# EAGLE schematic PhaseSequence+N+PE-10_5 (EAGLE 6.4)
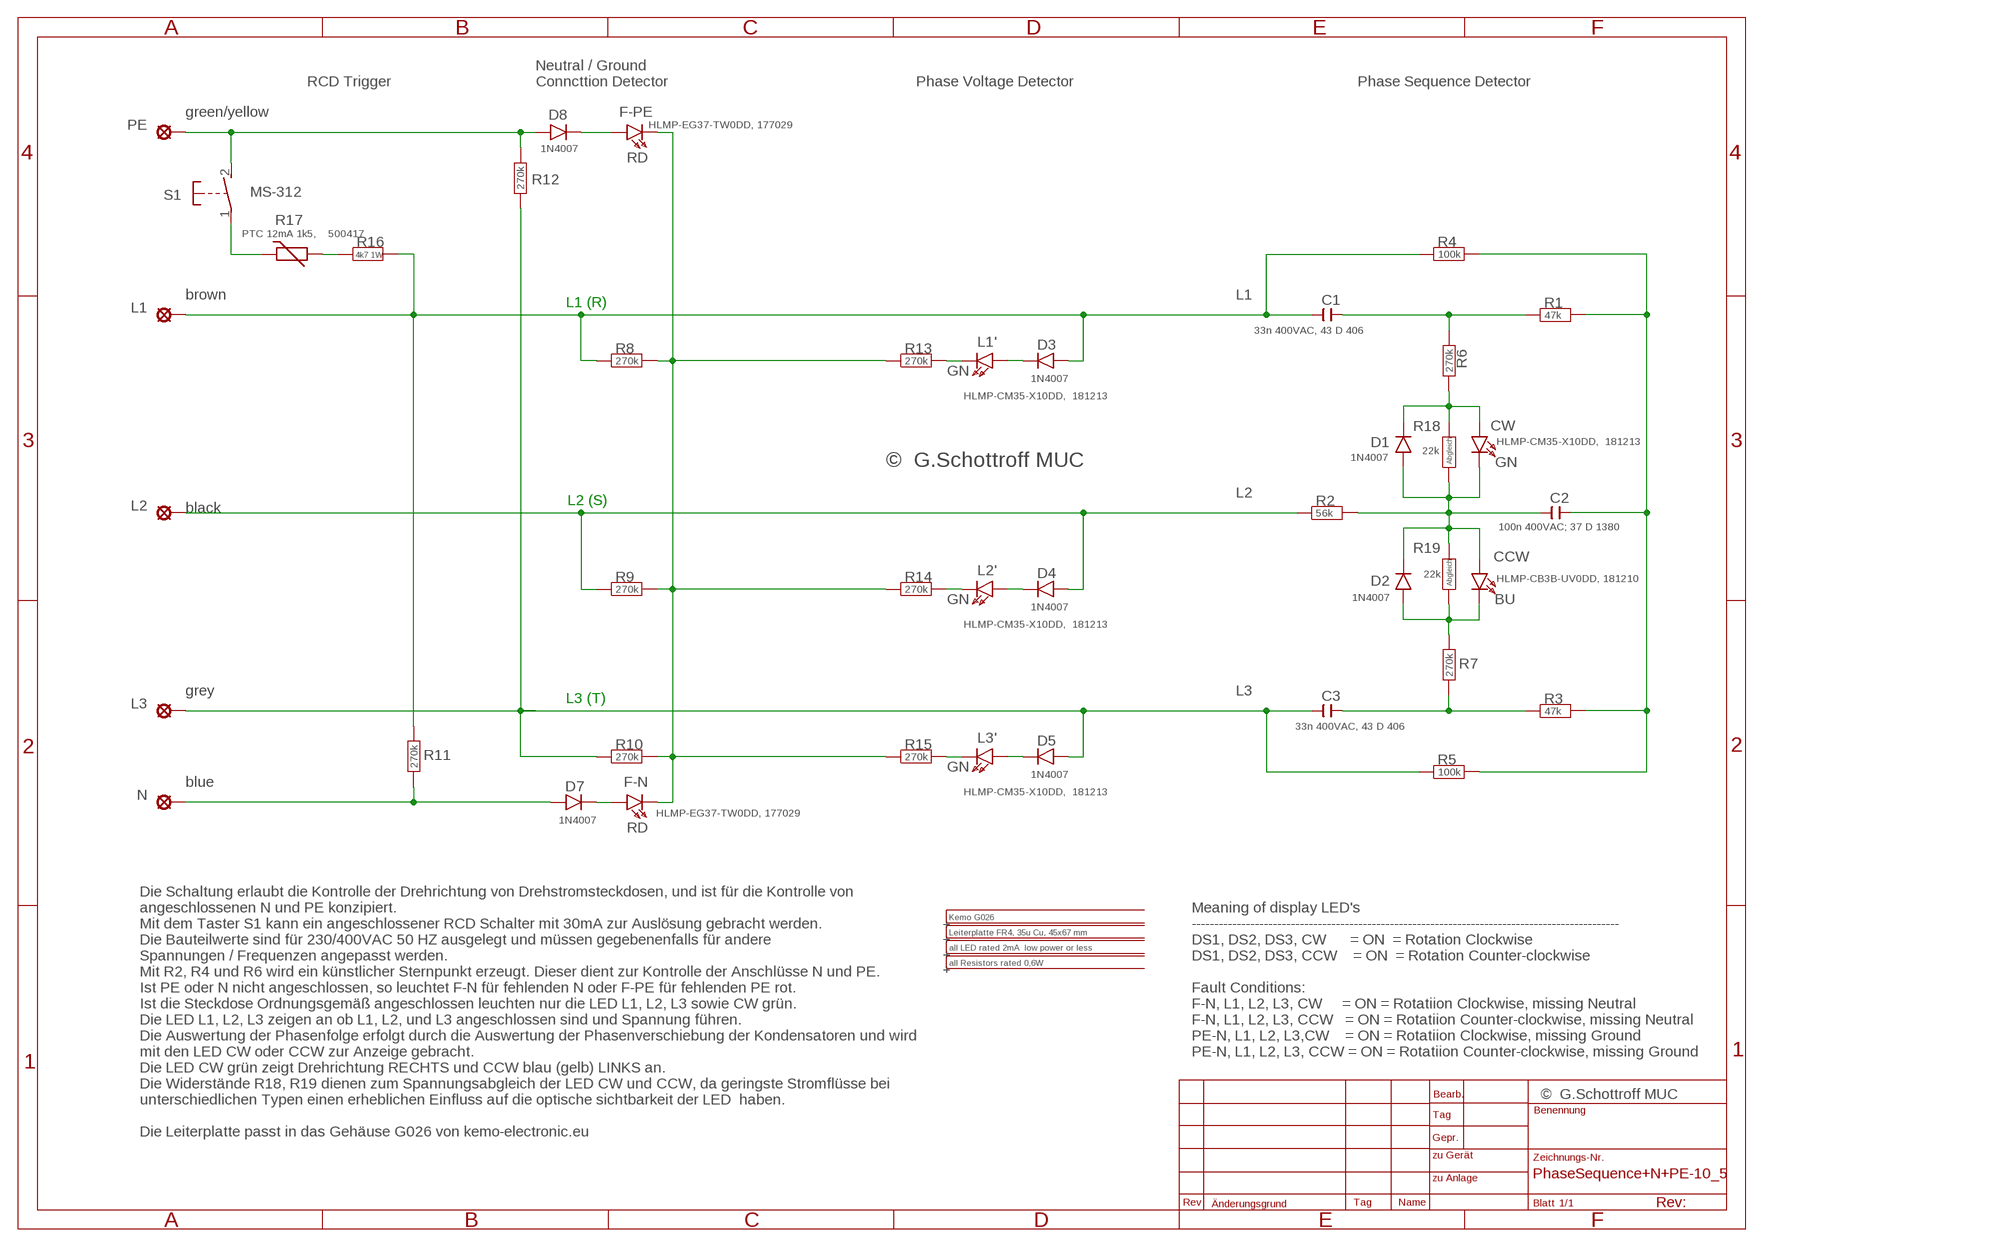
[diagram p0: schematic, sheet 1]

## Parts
C1  33n 400VAC, 43 D 406  C-EU150-064X183  [C150-064X183]
C2  100n 400VAC; 37 D 1380  C-EU150-084X183  [C150-084X183]
C3  33n 400VAC, 43 D 406  C-EU150-064X183  [C150-064X183]
CCW  HLMP-CB3B-UV0DD, 181210  LED5MM  [LED5MM]
CW  HLMP-CM35-X10DD, 181213  LED5MM  [LED5MM]
D1  1N4007  1N4004  [DO41-10]
D2  1N4007  1N4004  [DO41-10]
D3  1N4007  1N4004  [DO41-10]
D4  1N4007  1N4004  [DO41-10]
D5  1N4007  1N4004  [DO41-10]
D7  1N4007  1N4004  [DO41-10]
D8  1N4007  1N4004  [DO41-10]
ENCLOSURE-1  Kemo G026  KEMO-G025  [KEMO-G025]
F-N  HLMP-EG37-TW0DD, 177029  LED5MM  [LED5MM]
F-PE  HLMP-EG37-TW0DD, 177029  LED5MM  [LED5MM]
INFO  all Resistors rated 0,6W  INFO  [INFO]
INFO1  all LED rated 2mA low power or less  INFO  [INFO]
L1  SE13  [SE13]
L1'  HLMP-CM35-X10DD, 181213  LED5MM  [LED5MM]
L2  SE13  [SE13]
L2'  HLMP-CM35-X10DD, 181213  LED5MM  [LED5MM]
L3  SE13  [SE13]
L3'  HLMP-CM35-X10DD, 181213  LED5MM  [LED5MM]
N  SE13  [SE13]
PCB  Leiterplatte FR4, 35u Cu, 45x67 mm  INFO  [INFO]
PE  SE13  [SE13]
R1  47k  R-EU_0207/10  [0207/10]
R2  56k  R-EU_0207/10  [0207/10]
R3  47k  R-EU_0207/10  [0207/10]
R4  100k  R-EU_0207/10  [0207/10]
R5  100k  R-EU_0207/10  [0207/10]
R6  270k  R-EU_0207/10  [0207/10]
R7  270k  R-EU_0207/10  [0207/10]
R8  270k  R-EU_0207/10  [0207/10]
R9  270k  R-EU_0207/10  [0207/10]
R10  270k  R-EU_0207/10  [0207/10]
R11  270k  R-EU_0207/10  [0207/10]
R12  270k  R-EU_0207/10  [0207/10]
R13  270k  R-EU_0207/10  [0207/10]
R14  270k  R-EU_0207/10  [0207/10]
R15  270k  R-EU_0207/10  [0207/10]
R16  4k7 1W  R-EU_0817/22  [P0817/22]
R17  PTC 12mA 1k5, 500417  THERMISTOR-5  [R-5]
R18  22k  R-EU_R1206  [1206]
R19  22k  R-EU_R1206  [1206]
S1  MS-312  [MS-312]

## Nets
L1: C1.2 D3.A L1.MP R4.1 R8.1 R11.2 R16.2
L2: D4.A L2.MP R2.1 R9.1
L3: C3.2 D5.A L3.MP R5.1 R10.1 R12.2
N$1: C3.1 R3.1 R7.1
N$2: C2.2 CCW.A CW.K(C) D1.A D2.C R2.2 R18.1 R19.2
N$3: C1.1 R1.1 R6.1
N$4: C2.1 R1.2 R3.2 R4.2 R5.2
N$5: CCW.K(C) D2.A R7.2 R19.1
N$6: CW.A D1.C R6.2 R18.2
N$7: F-N.K(C) F-PE.K(C) R8.2 R9.2 R10.2 R13.1 R14.1 R15.1
N$8: D7.A N.MP R11.1
N$9: L1'.K(C) R13.2
N$10: L2'.K(C) R14.2
N$11: D7.C F-N.A
N$12: D8.A PE.MP R12.1 S1.2(S)
N$13: D8.C F-PE.A
N$14: L3'.K(C) R15.2
N$15: R17.1 S1.1(P)
N$16: D3.C L1'.A
N$17: R16.1 R17.2
N$18: D4.C L2'.A
N$19: D5.C L3'.A

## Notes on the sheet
- RCD Trigger
- Neutral / Ground 
  Conncttion Detector
- Phase Voltage Detector | Phase Sequence Detector
- green/yellow
- RD
- brown
- L1 (R)
- GN
- Abgleich
- ©  G.Schottroff MUC | GN
- L2 (S)
- black
- Abgleich
- GN | BU
- grey
- L3 (T)
- GN
- blue
- RD
- Meaning of display LED's
  -----------------------------------------------------------------------------------------------
  DS1, DS2, DS3, CW      = ON  = Rotation Clockwise
  DS1, DS2, DS3, CCW    = ON  = Rotation Counter-clockwise
  
  Fault Conditions:
  F-N, L1, L2, L3, CW     = ON = Rotatiion Clockwise, missing Neutral
  F-N, L1, L2, L3, CCW   = ON = Rotatiion Counter-clockwise, missing Neutral
  PE-N, L1, L2, L3,CW    = ON = Rotatiion Clockwise, missing Ground
  PE-N, L1, L2, L3, CCW = ON = Rotatiion Counter-clockwise, missing Ground
- ©  G.Schottroff MUC
- Die Schaltung erlaubt die Kontrolle der Drehrichtung von Drehstromsteckdosen, und ist für die Kontrolle von 
  angeschlossenen N und PE konzipiert. 
  Mit dem Taster S1 kann ein angeschlossener RCD Schalter mit 30mA zur Auslösung gebracht werden.
  Die Bauteilwerte sind für 230/400VAC 50 HZ ausgelegt und müssen gegebenenfalls für andere 
  Spannungen / Frequenzen angepasst werden.
  Mit R2, R4 und R6 wird ein künstlicher Sternpunkt erzeugt. Dieser dient zur Kontrolle der Anschlüsse N und PE. 
  Ist PE oder N nicht angeschlossen, so leuchtet F-N für fehlenden N oder F-PE für fehlenden PE rot.
  Ist die Steckdose Ordnungsgemäß angeschlossen leuchten nur die LED L1, L2, L3 sowie CW grün.
  Die LED L1, L2, L3 zeigen an ob L1, L2, und L3 angeschlossen sind und Spannung führen.
  Die Auswertung der Phasenfolge erfolgt durch die Auswertung der Phasenverschiebung der Kondensatoren und wird 
  mit den LED CW oder CCW zur Anzeige gebracht.
  Die LED CW grün zeigt Drehrichtung RECHTS und CCW blau (gelb) LINKS an.
  Die Widerstände R18, R19 dienen zum Spannungsabgleich der LED CW und CCW, da geringste Stromflüsse bei 
  unterschiedlichen Typen einen erheblichen Einfluss auf die optische sichtbarkeit der LED  haben.
  
  Die Leiterplatte passt in das Gehäuse G026 von kemo-electronic.eu

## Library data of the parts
C1-C3 = rcl:C-EU: CAPACITOR, European symbol
CCW CW F-N F-PE L1' L2' L3' = led:LED: LED
D1-D5 D7 D8 = diode:1N4004: DIODE
ENCLOSURE-1 = Enclosures-DIN-Rail+more:KEMO-G025
INFO INFO1 PCB = frames:INFO
L1-L3 N PE = solpad:SE13: SOLDER PAD
R1-R16 R18 R19 = rcl:R-EU_: RESISTOR, European symbol
R17 = varistor:THERMISTOR: THERMISTOR
S1 = switch-misc:MS-312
